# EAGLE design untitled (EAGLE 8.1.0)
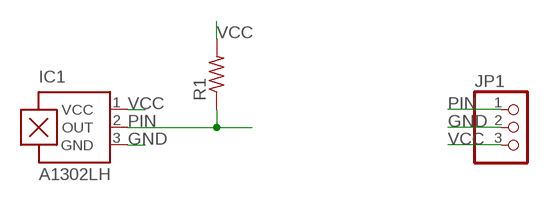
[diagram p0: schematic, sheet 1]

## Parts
IC1  A1302LH  [SOT23-W]
JP1  PINHD-1X3  [1X03]
R1  RES-US1206FAB  [R1206FAB]

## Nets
GND: IC1.3(GND) JP1.2
PIN: IC1.2(OUT) JP1.1 R1.1
VCC: IC1.1(VCC) JP1.3 R1.2

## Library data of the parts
IC1 = allegro:A13*?: Linear Hall Effect Sensor ICs Continuous-Time Ratiometric High-Temperature Operation Programmable Linear with Analog Output A1302 -Replacement- UGN3503 Source: http://www.allegromicro.com/en/Products/Part_Numbers/1301/1301.pdf http://www.allegromicro.com/en/Products/Part_Numbers/1321/1321.pdf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; MF: ALLEGRO MICROSYSTEMS, INC.; MPN: A1302ELHLT-T; OC_FARNELL: 1457209; OC_NEWARK: 31K6638
JP1 = adafruit:PINHD-1X3: PIN HEADER
R1 = fab:RES-US: Resistor (US Symbol)

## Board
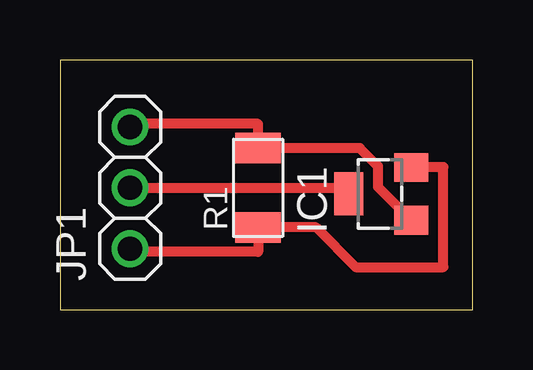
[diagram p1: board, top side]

Size 17.2 x 10.4 mm. Coordinates in mm from the lower left corner, seen from the top.
Outline: 0,0 17.2,0 17.2,10.4 0,10.4 0,0
Copper layers (1*16): Top 0.035mm / dielectric 1.5mm / Bottom 0.035mm
Design rules "default *": minimum track width 10mil, minimum drill 24mil, track to track 16mil, track to pad 16mil, pad to pad 16mil, via to via 16mil, smd to smd 16mil, copper to edge 40mil, drill to drill 8mil, minimum pad ring 10mil, minimum via ring 8mil, stop-mask expansion 4mil, vias tented up to drill 0mil, thermal gap 10mil

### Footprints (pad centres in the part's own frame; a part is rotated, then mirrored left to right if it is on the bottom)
SOT23-W = smd 1.2 x 1.4: 1 -1.1,-1.3; 2 1.1,-1.3 | smd 1.8 x 1.2: 3 0,1.3
1X03 = drill 1.016: 1 -2.54,0; 2 0,0; 3 2.54,0
R1206FAB = smd 1.27 x 1.905: 1 -1.651,0; 2 1.651,0

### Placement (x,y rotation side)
IC1  13.33,4.83 90 top
JP1  2.92,5.08 90 top
R1  8.25,5.08 90 top

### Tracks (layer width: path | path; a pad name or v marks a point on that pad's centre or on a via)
GND
  Top 0.406: 11.79,5.07 IC1.3 11.78,5.08 JP1.2
PIN
  Top 0.406: IC1.2 14.65,5.94 15.98,5.94 15.98,1.78 12.32,1.78 10.67,3.43 R1.1 8.25,2.41 3.05,2.41 JP1.1
VCC
  Top 0.406: IC1.1 13.24,5.12 13.24,5.98 12.49,6.73 R1.2 8.25,7.75 3.05,7.75 JP1.3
